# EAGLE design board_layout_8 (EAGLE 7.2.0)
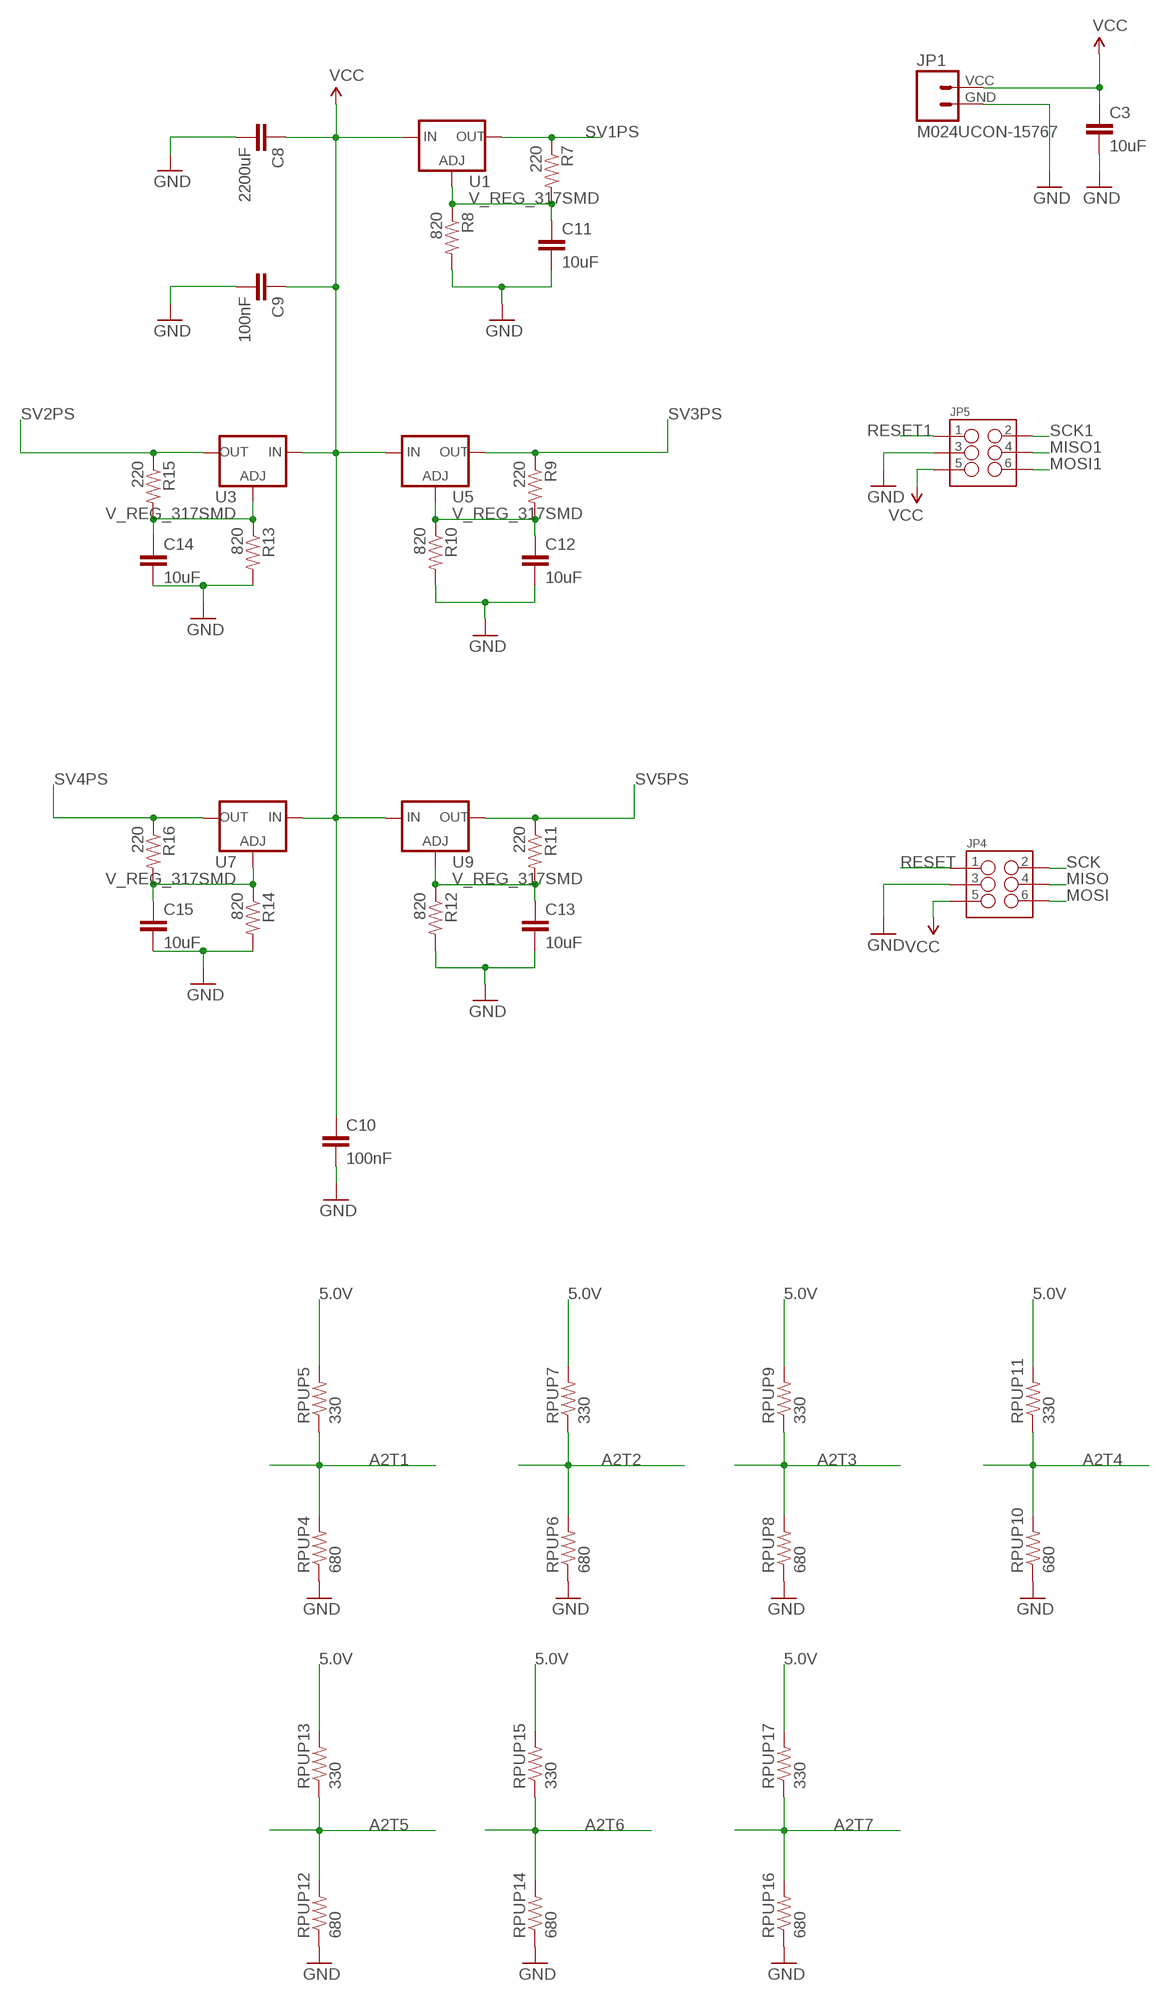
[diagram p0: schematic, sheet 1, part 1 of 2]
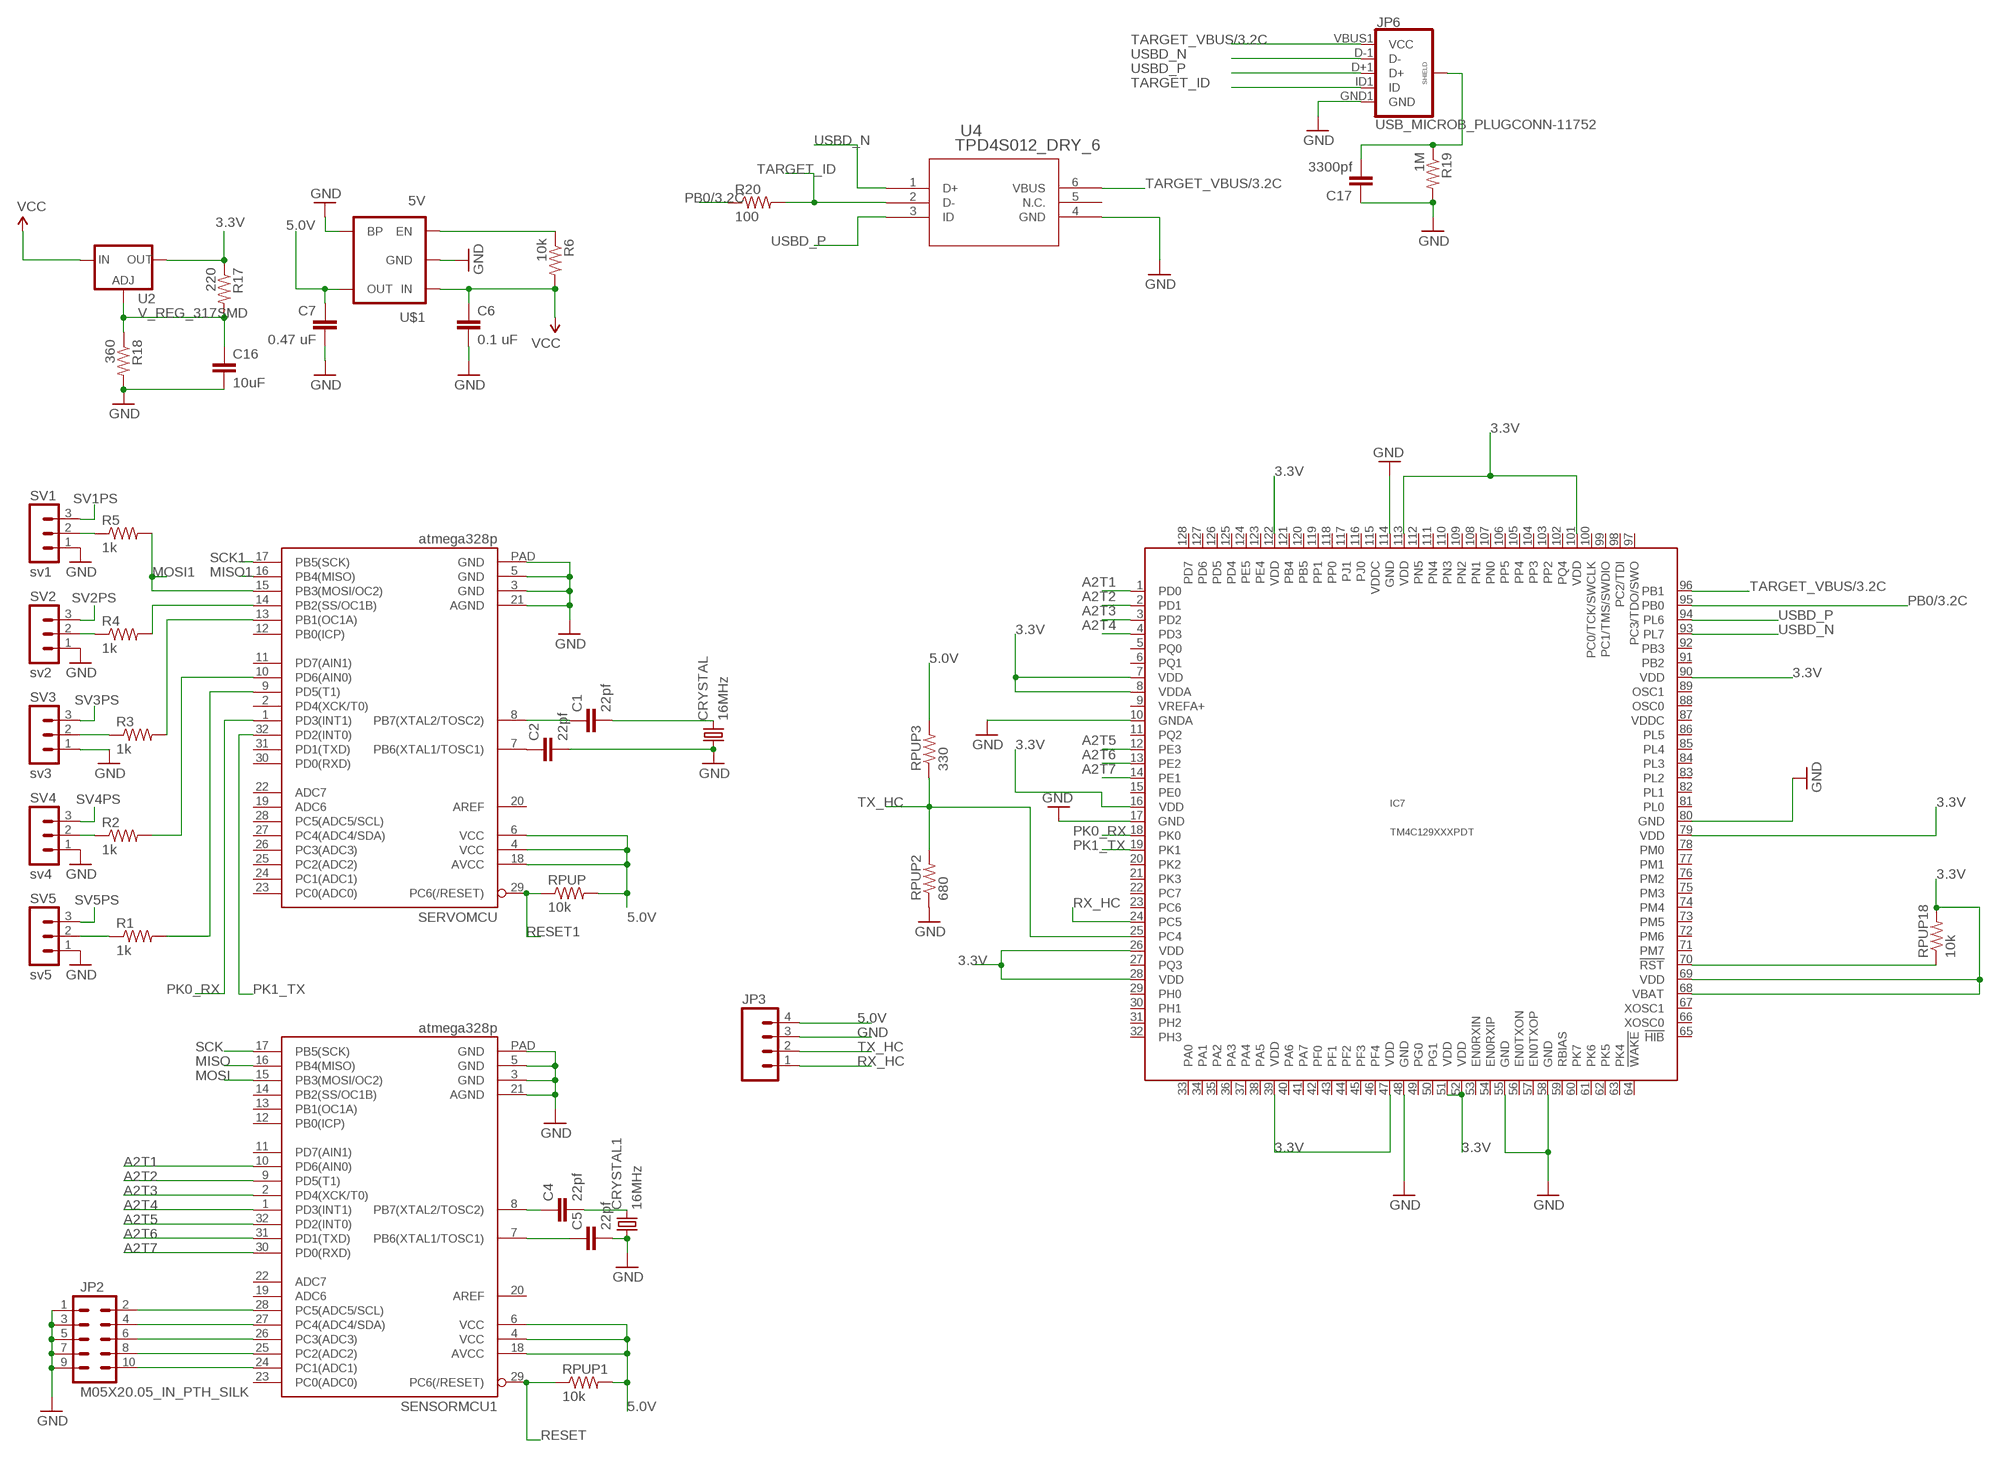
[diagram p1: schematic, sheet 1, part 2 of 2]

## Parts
C1  22pf  CAP0402-CAP  [0402-CAP]
C2  22pf  CAP0402-CAP  [0402-CAP]
C3  10uF  CAP0805  [0805]
C4  22pf  CAP0402-CAP  [0402-CAP]
C5  22pf  CAP0402-CAP  [0402-CAP]
C6  0.1 uF  CAP0805  [0805]
C7  0.47 uF  CAP0805  [0805]
C8  2200uF  CAP0805  [0805]
C9  100nF  CAP0805  [0805]
C10  100nF  CAP0805  [0805]
C11  10uF  CAP0805  [0805]
C12  10uF  CAP0805  [0805]
C13  10uF  CAP0805  [0805]
C14  10uF  CAP0805  [0805]
C15  10uF  CAP0805  [0805]
C16  10uF  CAP0805  [0805]
C17  3300pf  CAP0402-CAP  [0402-CAP]
CRYSTAL  16MHz  CRYSTALTC26V  [TC26V]
CRYSTAL1  16MHz  CRYSTALTC26V  [TC26V]
IC7  TM4C129XXXPDT  [PDT_S-PQFP-G128]
JP1  M024UCON-15767  [JST-2-SMD-VERT]
JP2  M05X20.05_IN_PTH_SILK  [2X5_PTH_SILK_.05]
JP3  M04SMD  [1X04-SMD]
JP4  M03X2  [2X3_SMD]
JP5  M03X2  [2X3_SMD]
JP6  USB_MICROB_PLUGCONN-11752  [USB-B-MICRO-SMD_V03]
R1  1k  RESISTOR0402-RES  [0402-RES]
R2  1k  RESISTOR0402-RES  [0402-RES]
R3  1k  RESISTOR0402-RES  [0402-RES]
R4  1k  RESISTOR0402-RES  [0402-RES]
R5  1k  RESISTOR0402-RES  [0402-RES]
R6  10k  RESISTOR0805-RES  [0805]
R7  220  RESISTOR0805-RES  [0805]
R8  820  RESISTOR0805-RES  [0805]
R9  220  RESISTOR0805-RES  [0805]
R10  820  RESISTOR0805-RES  [0805]
R11  220  RESISTOR0805-RES  [0805]
R12  820  RESISTOR0805-RES  [0805]
R13  820  RESISTOR0805-RES  [0805]
R14  820  RESISTOR0805-RES  [0805]
R15  220  RESISTOR0805-RES  [0805]
R16  220  RESISTOR0805-RES  [0805]
R17  220  RESISTOR0805-RES  [0805]
R18  360  RESISTOR0805-RES  [0805]
R19  1M  RESISTOR0805-RES  [0805]
R20  100  RESISTOR0805-RES  [0805]
RPUP  10k  RESISTOR0402-RES  [0402-RES]
RPUP1  10k  RESISTOR0402-RES  [0402-RES]
RPUP2  680  RESISTOR0402-RES  [0402-RES]
RPUP3  330  RESISTOR0402-RES  [0402-RES]
RPUP4  680  RESISTOR0402-RES  [0402-RES]
RPUP5  330  RESISTOR0402-RES  [0402-RES]
RPUP6  680  RESISTOR0402-RES  [0402-RES]
RPUP7  330  RESISTOR0402-RES  [0402-RES]
RPUP8  680  RESISTOR0402-RES  [0402-RES]
RPUP9  330  RESISTOR0402-RES  [0402-RES]
RPUP10  680  RESISTOR0402-RES  [0402-RES]
RPUP11  330  RESISTOR0402-RES  [0402-RES]
RPUP12  680  RESISTOR0402-RES  [0402-RES]
RPUP13  330  RESISTOR0402-RES  [0402-RES]
RPUP14  680  RESISTOR0402-RES  [0402-RES]
RPUP15  330  RESISTOR0402-RES  [0402-RES]
RPUP16  680  RESISTOR0402-RES  [0402-RES]
RPUP17  330  RESISTOR0402-RES  [0402-RES]
RPUP18  10k  RESISTOR0402-RES  [0402-RES]
SENSORMCU1  atmega328p  ATMEGA328P_MLFMLF32  [MLF32-PAD]
SERVOMCU  atmega328p  ATMEGA328P_MLFMLF32  [MLF32-PAD]
SV1  sv1  MA03-1  [MA03-1]
SV2  sv2  MA03-1  [MA03-1]
SV3  sv3  MA03-1  [MA03-1]
SV4  sv4  MA03-1  [MA03-1]
SV5  sv5  MA03-1  [MA03-1]
U1  V_REG_317SMD  [SOT223]
U2  V_REG_317SMD  [SOT223]
U3  V_REG_317SMD  [SOT223]
U4  TPD4S012_DRY_6  [DRY6]
U5  V_REG_317SMD  [SOT223]
U7  V_REG_317SMD  [SOT223]
U9  V_REG_317SMD  [SOT223]
U$1  5V  V_REG_MIC52055V  [SOT23-5]

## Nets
3.3V: IC7.7(VDD) IC7.8(VDDA) IC7.16(VDD) IC7.26(VDD) IC7.28(VDD) IC7.39(VDD) IC7.47(VDD) IC7.51(VDD) IC7.52(VDD) IC7.68(VBAT) IC7.69(VDD) IC7.79(VDD) IC7.90(VDD) IC7.101(VDD) IC7.113(VDD) IC7.122(VDD) R17.1 RPUP18.2 U2.2(OUT)
5.0V: C7.1 JP3.4 RPUP1.2 RPUP3.2 RPUP5.2 RPUP7.2 RPUP9.2 RPUP11.2 RPUP13.2 RPUP15.2 RPUP17.2 RPUP.2 SENSORMCU1.4(VCC) SENSORMCU1.6(VCC) SENSORMCU1.18(AVCC) SERVOMCU.4(VCC) SERVOMCU.6(VCC) SERVOMCU.18(AVCC) U$1.5(OUT)
A2T1: IC7.1(PD0) RPUP4.2 RPUP5.1 SENSORMCU1.10(PD6(AIN0))
A2T2: IC7.2(PD1) RPUP6.2 RPUP7.1 SENSORMCU1.9(PD5(T1))
A2T3: IC7.3(PD2) RPUP8.2 RPUP9.1 SENSORMCU1.2(PD4(XCK/T0))
A2T4: IC7.4(PD3) RPUP10.2 RPUP11.1 SENSORMCU1.1(PD3(INT1))
A2T5: IC7.12(PE3) RPUP12.2 RPUP13.1 SENSORMCU1.32(PD2(INT0))
A2T6: IC7.13(PE2) RPUP14.2 RPUP15.1 SENSORMCU1.31(PD1(TXD))
A2T7: IC7.14(PE1) RPUP16.2 RPUP17.1 SENSORMCU1.30(PD0(RXD))
GND: C2.2 C3.2 C5.2 C6.2 C7.2 C8.2 C9.2 C10.2 C11.2 C12.2 C13.2 C14.2 C15.2 C16.2 C17.1 CRYSTAL1.1 CRYSTAL.1 IC7.10(GNDA) IC7.17(GND) IC7.48(GND) IC7.55(GND) IC7.58(GND) IC7.80(GND) IC7.114(GND) JP1.GND JP2.1 JP2.3 JP2.5 JP2.7 JP2.9 JP3.3 JP4.3 JP5.3 JP6.GND1(GND) R8.2 R10.2 R12.2 R13.2 R14.2 R18.2 R19.2 RPUP2.1 RPUP4.1 RPUP6.1 RPUP8.1 RPUP10.1 RPUP12.1 RPUP14.1 RPUP16.1 SENSORMCU1.3(GND) SENSORMCU1.5(GND) SENSORMCU1.21(AGND) SENSORMCU1.PAD(GND) SERVOMCU.3(GND) SERVOMCU.5(GND) SERVOMCU.21(AGND) SERVOMCU.PAD(GND) SV1.1 SV2.1 SV3.1 SV4.1 SV5.1 U4.4(GND) U$1.2(GND) U$1.4(BP)
MISO: JP4.4 SENSORMCU1.16(PB4(MISO))
MISO1: JP5.4 SERVOMCU.16(PB4(MISO))
MOSI: JP4.6 SENSORMCU1.15(PB3(MOSI/OC2))
MOSI1: JP5.6 R5.2 SERVOMCU.15(PB3(MOSI/OC2))
N$1: R6.1 U$1.3(EN)
N$2: R4.2 SERVOMCU.14(PB2(SS/OC1B))
N$3: R3.2 SERVOMCU.13(PB1(OC1A))
N$4: C11.1 R7.2 R8.1 U1.1(ADJ)
N$5: R2.1 SV4.2
N$6: R1.1 SV5.2
N$7: R2.2 SERVOMCU.10(PD6(AIN0))
N$8: R1.2 SERVOMCU.9(PD5(T1))
N$9: R3.1 SV3.2
N$10: C1.1 SERVOMCU.8(PB7(XTAL2/TOSC2))
N$11: C2.1 SERVOMCU.7(PB6(XTAL1/TOSC1))
N$12: R5.1 SV1.2
N$13: R4.1 SV2.2
N$14: C16.1 R17.2 R18.1 U2.1(ADJ)
N$15: JP2.10 SENSORMCU1.24(PC1(ADC1))
N$16: JP2.8 SENSORMCU1.25(PC2(ADC2))
N$17: C4.1 SENSORMCU1.8(PB7(XTAL2/TOSC2))
N$18: C4.2 CRYSTAL1.2
N$19: C5.1 SENSORMCU1.7(PB6(XTAL1/TOSC1))
N$20: C1.2 CRYSTAL.2
N$21: JP2.6 SENSORMCU1.26(PC3(ADC3))
N$22: JP2.4 SENSORMCU1.27(PC4(ADC4/SDA))
N$23: JP2.2 SENSORMCU1.28(PC5(ADC5/SCL))
N$25: C12.1 R9.2 R10.1 U5.1(ADJ)
N$26: C13.1 R11.2 R12.1 U9.1(ADJ)
N$29: C14.1 R13.1 R15.2 U3.1(ADJ)
N$31: C15.1 R14.1 R16.2 U7.1(ADJ)
N$38: C17.2 JP6.SHIELD1(SHIELD) JP6.SHIELD2(SHIELD) JP6.SHIELD3(SHIELD) R19.1
N$41: IC7.70(!RST) RPUP18.1
PB0/3.2C: IC7.95(PB0) R20.1
PK0_RX: IC7.18(PK0) SERVOMCU.1(PD3(INT1))
PK1_TX: IC7.19(PK1) SERVOMCU.32(PD2(INT0))
RESET: JP4.1 RPUP1.1 SENSORMCU1.29(PC6(/RESET))
RESET1: JP5.1 RPUP.1 SERVOMCU.29(PC6(/RESET))
RX_HC: IC7.24(PC5) JP3.1
SCK: JP4.2 SENSORMCU1.17(PB5(SCK))
SCK1: JP5.2 SERVOMCU.17(PB5(SCK))
SV1PS: R7.1 SV1.3 U1.2(OUT)
SV2PS: R15.1 SV2.3 U3.2(OUT)
SV3PS: R9.1 SV3.3 U5.2(OUT)
SV4PS: R16.1 SV4.3 U7.2(OUT)
SV5PS: R11.1 SV5.3 U9.2(OUT)
TARGET_ID: JP6.ID1(ID) R20.2 U4.2(D-)
TARGET_VBUS/3.2C: IC7.96(PB1) JP6.VBUS1(VCC) U4.6(VBUS)
TX_HC: IC7.25(PC4) JP3.2 RPUP2.2 RPUP3.1
USBD_N: IC7.93(PL7) JP6.D-1(D-) U4.1(D+)
USBD_P: IC7.94(PL6) JP6.D+1(D+) U4.3(ID)
VCC: C3.1 C6.1 C8.1 C9.1 C10.1 JP1.VCC JP4.5 JP5.5 R6.2 U1.3(IN) U2.3(IN) U3.3(IN) U5.3(IN) U7.3(IN) U9.3(IN) U$1.1(IN)
Unconnected: IC7.5(PQ0) IC7.6(PQ1) IC7.9(VREFA+) IC7.11(PQ2) IC7.15(PE0) IC7.20(PK2) IC7.21(PK3) IC7.22(PC7) IC7.23(PC6) IC7.27(PQ3) IC7.29(PH0) IC7.30(PH1) IC7.31(PH2) IC7.32(PH3) IC7.33(PA0) IC7.34(PA1) IC7.35(PA2) IC7.36(PA3) IC7.37(PA4) IC7.38(PA5) IC7.40(PA6) IC7.41(PA7) IC7.42(PF0) IC7.43(PF1) IC7.44(PF2) IC7.45(PF3) IC7.46(PF4) IC7.49(PG0) IC7.50(PG1) IC7.53(EN0RXIN) IC7.54(EN0RXIP) IC7.56(EN0TXON) IC7.57(EN0TXOP) IC7.59(RBIAS) IC7.60(PK7) IC7.61(PK6) IC7.62(PK5) IC7.63(PK4) IC7.64(!WAKE) IC7.65(!HIB) IC7.66(XOSC0) IC7.67(XOSC1) IC7.71(PM7) IC7.72(PM6) IC7.73(PM5) IC7.74(PM4) IC7.75(PM3) IC7.76(PM2) IC7.77(PM1) IC7.78(PM0) IC7.81(PL0) IC7.82(PL1) IC7.83(PL2) IC7.84(PL3) IC7.85(PL4) IC7.86(PL5) IC7.87(VDDC) IC7.88(OSC0) IC7.89(OSC1) IC7.91(PB2) IC7.92(PB3) IC7.97(PC3/TDO/SWO) IC7.98(PC2/TDI) IC7.99(PC1/TMS/SWDIO) IC7.100(PC0/TCK/SWCLK) IC7.102(PQ4) IC7.103(PP2) IC7.104(PP3) IC7.105(PP4) IC7.106(PP5) IC7.107(PN0) IC7.108(PN1) IC7.109(PN2) IC7.110(PN3) IC7.111(PN4) IC7.112(PN5) IC7.115(VDDC) IC7.116(PJ0) IC7.117(PJ1) IC7.118(PP0) IC7.119(PP1) IC7.120(PB5) IC7.121(PB4) IC7.123(PE4) IC7.124(PE5) IC7.125(PD4) IC7.126(PD5) IC7.127(PD6) IC7.128(PD7) SENSORMCU1.11(PD7(AIN1)) SENSORMCU1.12(PB0(ICP)) SENSORMCU1.13(PB1(OC1A)) SENSORMCU1.14(PB2(SS/OC1B)) SENSORMCU1.19(ADC6) SENSORMCU1.20(AREF) SENSORMCU1.22(ADC7) SENSORMCU1.23(PC0(ADC0)) SERVOMCU.2(PD4(XCK/T0)) SERVOMCU.11(PD7(AIN1)) SERVOMCU.12(PB0(ICP)) SERVOMCU.19(ADC6) SERVOMCU.20(AREF) SERVOMCU.22(ADC7) SERVOMCU.23(PC0(ADC0)) SERVOMCU.24(PC1(ADC1)) SERVOMCU.25(PC2(ADC2)) SERVOMCU.26(PC3(ADC3)) SERVOMCU.27(PC4(ADC4/SDA)) SERVOMCU.28(PC5(ADC5/SCL)) SERVOMCU.30(PD0(RXD)) SERVOMCU.31(PD1(TXD)) U4.5(N.C.)

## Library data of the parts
C1 C2 C4-C7 C17 = SparkFun-Passives:CAP: Capacitor
C3 C8-C16 = SparkFun-Capacitors:CAP: Capacitor
CRYSTAL CRYSTAL1 = crystal:CRYSTAL: CRYSTAL; OC_FARNELL: unknown; OC_NEWARK: unknown
IC7 = ti-tiva:TM4C129XXX
JP1 = SparkFun-Connectors:M02: Standard 2-pin 0.1" header. Use with
JP2 = SparkFun-Connectors:M05X2: Header 5x2 Standard 10-pin dual row 0.1" header. Commonly used with AVR-ISP. Use with Spark Fun Electronics SKU: PRT-00778
JP3 = SparkFun-Connectors:M04: Header 4 Standard 4-pin 0.1" header. Use with straight break away headers (SKU : PRT-00116), right angle break away headers (PRT-00553), swiss pins (PRT-00743), machine pins (PRT-00117), and female headers (PRT-00115). Molex polarized connector foot print use with SKU : PRT-08231 with associated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
JP4 JP5 = SparkFun-Connectors:M03X2: 2x3 .1" header. Shrouded, with keying- CONN-10681 SMT- CONN-11415 Pogo pins- HW-11044; PROD_ID: CONN-11290
JP6 = SparkFun-Connectors:USB_MICROB_PLUG: USB Micro-B connectors Some male, some female. Watch your step!; PROD_ID: CONN-11752
R1-R20 RPUP RPUP1-RPUP18 = SparkFun-Passives:RESISTOR: Resistor
SENSORMCU1 SERVOMCU = SparkFun-DigitalIC:ATMEGA328P_MLF: 32-Pin Atmega328 part Commonly used on Arduino compatible boards Available in QFP and QFN packages TQFP is IC-09069 QFN is non-stock
SV1-SV5 = con-lstb:MA03-1: PIN HEADER; OC_FARNELL: unknown; OC_NEWARK: unknown
U1-U3 U5 U7 U9 = SparkFun-PowerIC:V_REG_317: Voltage Regulator Standard LM317 adjustable voltage regulator. AOI (Adjust Output Input). Google 'LM317 Calculator' for easy to use app to get the two resistor values needed. 240/720 for 5V output. 240/390 for 3.3V output. Spark Fun Electronics SKU : COM-00527
U4 = esd_tp:TPD4S012_DRY_6; DATASHEETURL: http://www.ti.com/lit/gpn/TPD4S012; DESCRIPTION: 4-Channel USB ESD Solution with Power Clamp; FAMILY_NAME: ESD Solution; GENERIC_PART_NUMBER: TPD4S012; INDUSTRY_STD_PKG_TYPE: SON; MANUFACTURER: Texas Instruments; MANUFACTURER_PART_NUMBER: tpd4s012_dry_6; PACKAGE_DESIGNATOR: DRY; PIN_COUNT: 6; VENDOR: Texas Instruments
U$1 = SparkFun-PowerIC:V_REG_MIC5205: V_REG MIC5219 Standard 3.3V and 5V 150mA LDO voltage regulator in SOT-23 layout. Micrel part MIC5205. BP (by-pass) pin is used to lower output noise with 470pF cap, may be left open.; PROD_ID: VREG-00823

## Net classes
0 default: clearance 0.06 mm

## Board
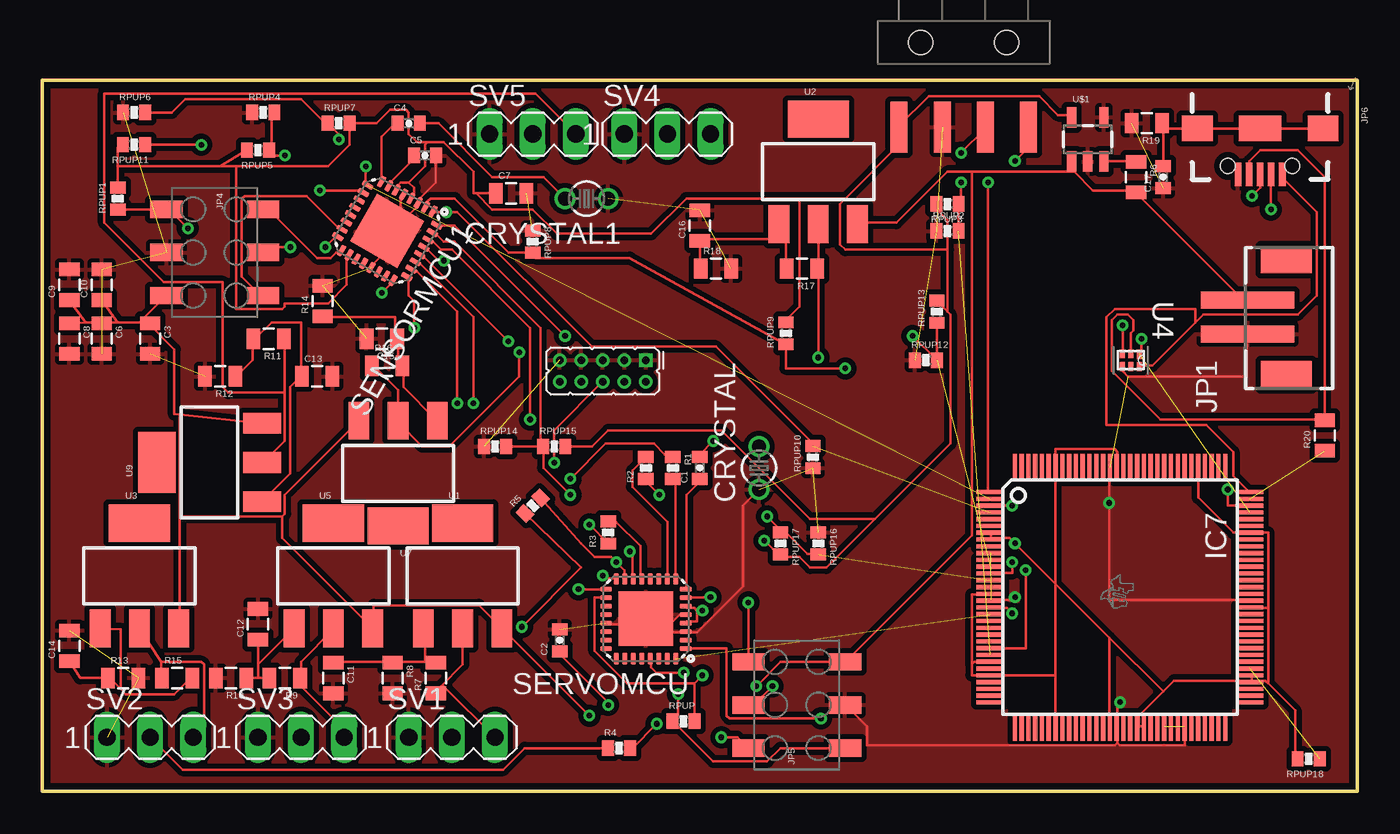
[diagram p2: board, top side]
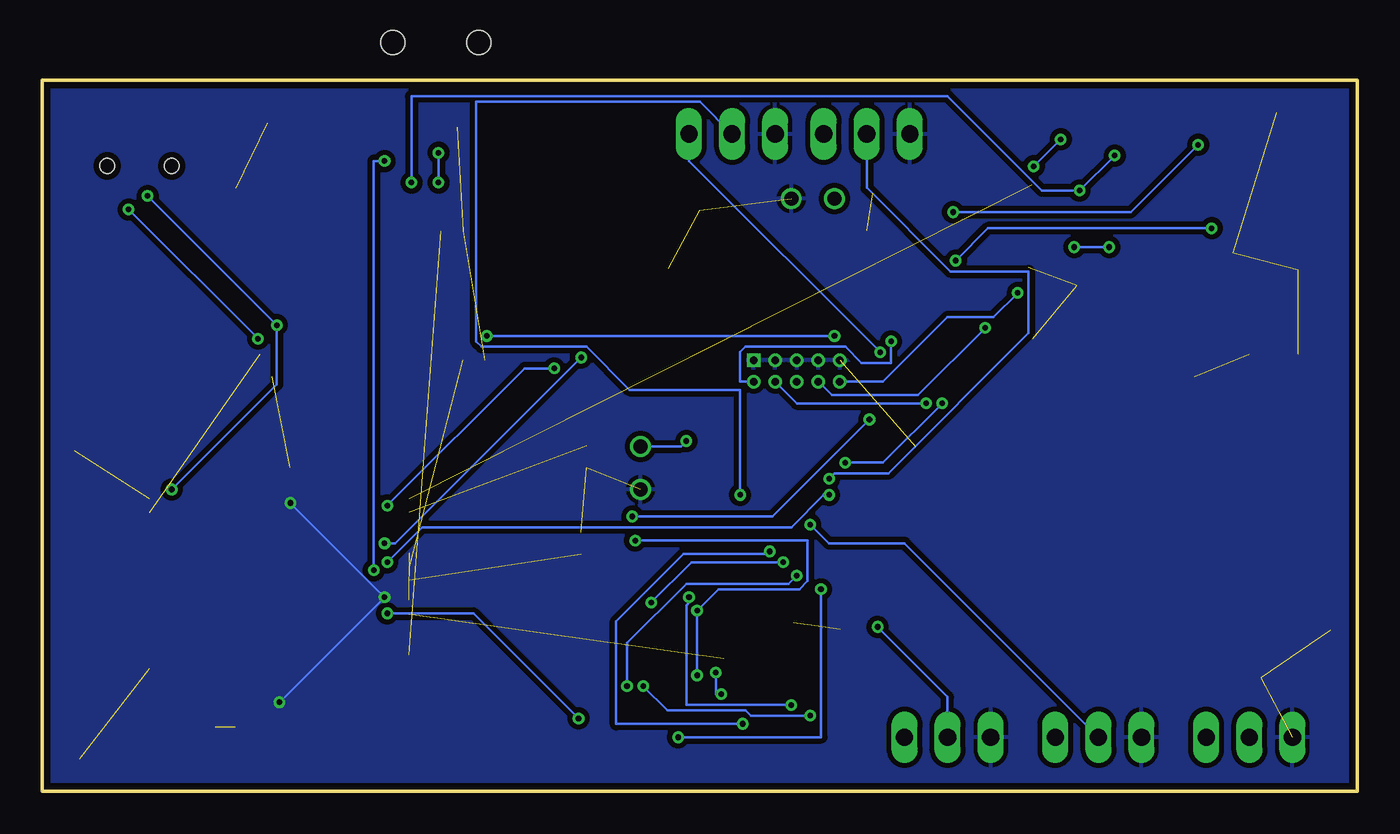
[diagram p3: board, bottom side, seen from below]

Size 77.47 x 41.91 mm. Coordinates in mm from the lower left corner, seen from the top.
Outline: 0,0 0,41.91 77.47,41.91 77.47,0 0,0
Copper layers (1*16): Top 0.0356mm / dielectric 1.5011mm / Bottom 0.0356mm
Design rules "PCB_order": minimum track width 6mil, minimum drill 13mil, track to track 6mil, track to pad 6mil, pad to pad 6mil, via to via 6mil, smd to smd 6mil, copper to edge 15mil, drill to drill 6mil, minimum pad ring 7mil, minimum via ring 7mil, stop-mask expansion 3mil, vias tented up to drill 0mil, thermal gap 10mil

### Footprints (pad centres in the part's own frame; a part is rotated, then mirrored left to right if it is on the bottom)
0402-CAP = smd 0.7 x 0.9: 1 -0.65,0; 2 0.65,0
0805 = smd 0.8 x 1.2: 1 -0.9,0; 2 0.9,0
TC26V = drill 0.813: 1 -1.27,0; 2 1.27,0
PDT_S-PQFP-G128 = smd 0.25 x 1.6: 1 -6.2,-7.65; 2 -5.8,-7.65; 3 -5.4,-7.65; 4 -5,-7.65; 5 -4.6,-7.65; 6 -4.2,-7.65; 7 -3.8,-7.65; 8 -3.4,-7.65; 9 -3,-7.65; 10 -2.6,-7.65; 11 -2.2,-7.65; 12 -1.8,-7.65; 13 -1.4,-7.65; 14 -1,-7.65; 15 -0.6,-7.65; 16 -0.2,-7.65; 17 0.2,-7.65; 18 0.6,-7.65; 19 1,-7.65; 20 1.4,-7.65; 21 1.8,-7.65; 22 2.2,-7.65; 23 2.6,-7.65; 24 3,-7.65; 25 3.4,-7.65; 26 3.8,-7.65; 27 4.2,-7.65; 28 4.6,-7.65; 29 5,-7.65; 30 5.4,-7.65; 31 5.8,-7.65; 32 6.2,-7.65; 65 6.2,7.65; 66 5.8,7.65; 67 5.4,7.65; 68 5,7.65; 69 4.6,7.65; 70 4.2,7.65; 71 3.8,7.65; 72 3.4,7.65; 73 3,7.65; 74 2.6,7.65; 75 2.2,7.65; 76 1.8,7.65; 77 1.4,7.65; 78 1,7.65; 79 0.6,7.65; 80 0.2,7.65; 81 -0.2,7.65; 82 -0.6,7.65; 83 -1,7.65; 84 -1.4,7.65; 85 -1.8,7.65; 86 -2.2,7.65; 87 -2.6,7.65; 88 -3,7.65; 89 -3.4,7.65; 90 -3.8,7.65; 91 -4.2,7.65; 92 -4.6,7.65; 93 -5,7.65; 94 -5.4,7.65; 95 -5.8,7.65; 96 -6.2,7.65 | smd 1.6 x 0.25: 33 7.65,-6.2; 34 7.65,-5.8; 35 7.65,-5.4; 36 7.65,-5; 37 7.65,-4.6; 38 7.65,-4.2; 39 7.65,-3.8; 40 7.65,-3.4; 41 7.65,-3; 42 7.65,-2.6; 43 7.65,-2.2; 44 7.65,-1.8; 45 7.65,-1.4; 46 7.65,-1; 47 7.65,-0.6; 48 7.65,-0.2; 49 7.65,0.2; 50 7.65,0.6; 51 7.65,1; 52 7.65,1.4; 53 7.65,1.8; 54 7.65,2.2; 55 7.65,2.6; 56 7.65,3; 57 7.65,3.4; 58 7.65,3.8; 59 7.65,4.2; 60 7.65,4.6; 61 7.65,5; 62 7.65,5.4; 63 7.65,5.8; 64 7.65,6.2; 97 -7.65,6.2; 98 -7.65,5.8; 99 -7.65,5.4; 100 -7.65,5; 101 -7.65,4.6; 102 -7.65,4.2; 103 -7.65,3.8; 104 -7.65,3.4; 105 -7.65,3; 106 -7.65,2.6; 107 -7.65,2.2; 108 -7.65,1.8; 109 -7.65,1.4; 110 -7.65,1; 111 -7.65,0.6; 112 -7.65,0.2; 113 -7.65,-0.2; 114 -7.65,-0.6; 115 -7.65,-1; 116 -7.65,-1.4; 117 -7.65,-1.8; 118 -7.65,-2.2; 119 -7.65,-2.6; 120 -7.65,-3; 121 -7.65,-3.4; 122 -7.65,-3.8; 123 -7.65,-4.2; 124 -7.65,-4.6; 125 -7.65,-5; 126 -7.65,-5.4; 127 -7.65,-5.8; 128 -7.65,-6.2
JST-2-SMD-VERT = smd 1 x 5.5: GND 1,-2; VCC -1,-2 | smd 1.6 x 3: P$1 -3.4,0.27; P$2 3.4,0.27
2X5_PTH_SILK_.05 = drill 0.432 square: 1 0,6.35 | drill 0.432: 2 1.27,6.35; 3 0,5.08; 4 1.27,5.08; 5 0,3.81; 6 1.27,3.81; 7 0,2.54; 8 1.27,2.54; 9 0,1.27; 10 1.27,1.27
1X04-SMD = smd 1 x 3: 1 -3.81,5; 2 -1.27,5; 3 1.27,5; 4 3.81,5 | hole 1.4: -2.54,0; 2.54,0
2X3_SMD = smd 1.02 x 1.9: 1 -2.54,-2.85; 2 -2.54,2.85; 3 0,-2.85; 4 0,2.85; 5 2.54,-2.85; 6 2.54,2.85
USB-B-MICRO-SMD_V03 = smd 1.4 x 0.4: D+1 2.7,0; D-1 2.7,0.65; GND1 2.7,-1.3; ID1 2.7,-0.65; VBUS1 2.7,1.3 | smd 1.5 x 1.8: SHIELD1 0,3.7; SHIELD2 0,-3.7 | smd 1.5 x 2.5: SHIELD3 0,0 | hole 0.85: 2.2,1.9; 2.2,-1.9
0402-RES = smd 0.7 x 0.9: 1 -0.65,0; 2 0.65,0
MLF32-PAD = smd 0.7 x 0.3: 1 -2.35,1.75; 2 -2.35,1.25; 3 -2.35,0.75; 4 -2.35,0.25; 5 -2.35,-0.25; 6 -2.35,-0.75; 7 -2.35,-1.25; 8 -2.35,-1.75; 17 2.35,-1.75; 18 2.35,-1.25; 19 2.35,-0.75; 20 2.35,-0.25; 21 2.35,0.25; 22 2.35,0.75; 23 2.35,1.25; 24 2.35,1.75 | smd 0.3 x 0.7: 9 -1.75,-2.35; 10 -1.25,-2.35; 11 -0.75,-2.35; 12 -0.25,-2.35; 13 0.25,-2.35; 14 0.75,-2.35; 15 1.25,-2.35; 16 1.75,-2.35; 25 1.75,2.35; 26 1.25,2.35; 27 0.75,2.35; 28 0.25,2.35; 29 -0.25,2.35; 30 -0.75,2.35; 31 -1.25,2.35; 32 -1.75,2.35 | smd 3.2 x 3.2: PAD 0,0
MA03-1 = drill 1.016 long: 1 -2.54,0; 2 0,0; 3 2.54,0
SOT223 = smd 1.219 x 2.235: 1 -2.311,-3.099; 2 0,-3.099; 3 2.311,-3.099 | smd 3.6 x 2.2: 4 0,3.099
DRY6 = smd 0.559 x 0.305: 1 -0.355,0.5 | smd 0.508 x 0.305: 2 -0.37,0; 3 -0.37,-0.5; 4 0.37,-0.5; 5 0.37,0; 6 0.37,0.5
SOT23-5 = smd 0.55 x 1.2: 1 -0.95,-1.3; 2 0,-1.3; 3 0.95,-1.3; 4 0.95,1.3; 5 -0.95,1.3

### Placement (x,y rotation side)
C1  38.74,19.05 90 top
C2  30.48,8.89 90 top
C3  6.35,26.67 270 top
C4  21.59,39.37 0 top
C5  22.54,37.47 0 top
C6  3.49,26.67 270 top
C7  27.62,35.24 0 top
C8  1.59,26.67 270 top
C9  1.59,29.84 90 top
C10  3.49,29.84 90 top
C11  17.14,6.67 270 top
C12  12.7,9.84 90 top
C13  16.19,24.45 0 top
C14  1.59,8.57 90 top
C15  20,26.67 180 top
C16  38.74,33.34 90 top
C17  66.04,36.2 90 top
CRYSTAL  42.23,19.05 90 top
CRYSTAL1  32.07,34.92 180 top
IC7  63.5,11.43 270 top
JP1  73.02,27.94 270 top
JP2  29.21,25.4 270 top
JP3  54.29,44.13 180 top
JP4  10.16,31.75 270 top
JP5  44.45,5.08 90 top
JP6  71.75,39.05 270 top
R1  37.15,19.05 270 top
R2  35.56,19.05 90 top
R3  33.34,15.24 90 top
R4  33.97,2.54 0 top
R5  28.89,16.83 45 top
R6  64.45,36.2 270 top
R7  23.18,6.67 90 top
R8  20.64,6.67 270 top
R9  14.29,6.67 180 top
R10  11.11,6.67 180 top
R11  13.33,26.67 180 top
R12  10.48,24.45 180 top
R13  4.76,6.67 0 top
R14  16.51,28.89 90 top
R15  7.94,6.67 0 top
R16  20.32,25.08 0 top
R17  44.77,30.8 180 top
R18  39.69,30.8 0 top
R19  65.09,39.37 180 top
R20  75.56,20.95 90 top
RPUP  37.78,4.13 0 top
RPUP1  4.45,34.92 90 top
RPUP2  53.34,33.02 0 top
RPUP3  53.34,34.61 180 top
RPUP4  13.02,40.01 0 top
RPUP5  12.7,37.78 180 top
RPUP6  5.4,40.01 0 top
RPUP7  17.46,39.37 0 top
RPUP8  28.89,32.38 270 top
RPUP9  43.82,26.99 90 top
RPUP10  45.4,19.68 90 top
RPUP11  5.4,38.1 180 top
RPUP12  52.07,25.4 0 top
RPUP13  52.71,28.26 90 top
RPUP14  26.67,20.32 0 top
RPUP15  30.16,20.32 0 top
RPUP16  45.72,14.61 270 top
RPUP17  43.5,14.61 270 top
RPUP18  74.61,1.91 180 top
SENSORMCU1  20.32,33.02 240 top
SERVOMCU  35.56,10.16 180 top
SV1  24.13,3.17 0 top
SV2  6.35,3.17 0 top
SV3  15.24,3.17 0 top
SV4  36.83,38.73 0 top
SV5  28.89,38.73 0 top
U1  24.77,12.7 0 top
U2  45.72,36.51 0 top
U3  5.71,12.7 0 top
U4  64.14,25.4 270 top
U5  17.14,12.7 0 top
U7  20.95,18.73 180 top
U9  9.84,19.37 90 top
U$1  61.6,38.42 0 top

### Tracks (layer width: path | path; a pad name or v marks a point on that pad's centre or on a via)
3.3V  (via drill 0.33)
  Top 0.152: U2.2 45.72,30.8 | 72.23,6.35 72.07,6.51 71.28,6.51 | 72.23,6.35 73.82,4.76 73.82,1.91 RPUP18.2 | 64.61,3.81 64.61,4.45 66.04,5.87 | 66.04,5.87 66.67,6.51 71.12,6.51 IC7.68 71.28,6.51 | 55.88,14.92 56.99,14.92 v57.31,14.61 59.69,12.22 | 66.04,5.87 62.87,9.05 | 62.87,9.05 59.69,12.22 | v45.72,25.56 45.72,30.8 | 45.72,30.8 R17.1 | 54.77,7.46 54.77,6.83 55.72,6.83 IC7.28 55.88,6.83 59.69,6.83 | 54.77,7.46 54.93,7.62 55.72,7.62 IC7.26 | 54.77,7.46 54.77,11.59 55.72,11.59 IC7.16 | 55.88,14.92 55.88,15.24 IC7.7 | 55.88,14.92 IC7.8 | 64.61,3.81 64.93,3.81 IC7.52 | 64.61,3.81 IC7.51 | 59.69,12.22 59.69,6.83 | 59.69,6.83 59.69,3.81 IC7.39 | 59.69,12.22 59.69,19.05 IC7.122 59.69,19.21 59.69,20.16 63.18,20.16 63.34,20 63.34,19.21 IC7.113 | 62.87,9.05 62.87,3.81 IC7.47 | 71.28,6.51 71.28,6.83 IC7.69 | 72.23,10.79 71.28,10.79 IC7.79 | 72.23,6.35 72.23,10.79 | 72.23,10.79 72.23,15.24 71.28,15.24 IC7.90 71.12,15.24 70.17,15.24 68.1,17.3 68.1,19.05 IC7.101
  Bottom 0.152: v45.72,25.56 56.67,14.61 v57.31,14.61
5.0V  (via drill 0.33)
  Top 0.152: 4.45,36.83 4.45,37.94 4.6,38.1 RPUP11.2 | 4.45,36.83 RPUP1.2 | 4.45,36.83 10.48,36.83 | 10.48,36.83 11.43,36.83 | 11.43,36.83 16.83,36.83 18.1,38.1 18.1,39.37 RPUP7.2 19.68,39.37 20.48,40.16 21.43,40.16 21.59,40.01 21.59,38.73 22.07,38.26 22.7,38.26 | 10.48,36.83 RPUP5.2 | 21.59,35.88 21.11,35.88 20.95,35.72 20.95,35.56 SENSORMCU1.6 | 21.59,35.88 21.91,35.56 21.91,35.24 21.75,35.08 SENSORMCU1.4 | 25.56,35.24 26.51,34.29 28.89,34.29 30.32,32.86 35.88,32.86 37.94,34.92 44.61,34.92 | 25.56,35.24 C7.1 | 21.59,35.88 22.54,36.83 22.54,38.1 22.7,38.26 | 22.7,38.26 23.65,38.26 25.4,36.51 25.4,35.24 25.56,35.24 | U$1.5 60.64,39.85 59.85,39.85 58.74,40.96 52.23,40.96 50.48,39.21 JP3.4 50.48,38.1 47.31,34.92 | 43.5,13.81 44.61,13.81 45.24,13.18 46.2,13.18 49.05,16.03 | 49.05,16.03 53.5,20.48 53.5,28.1 53.34,28.26 | 53.34,28.26 52.71,28.89 RPUP13.2 | 53.34,28.26 53.34,31.91 | 53.34,31.91 53.34,33.66 52.71,34.29 52.71,34.61 RPUP3.2 | 47.31,34.92 46.99,34.61 46.99,32.23 47.31,31.91 53.34,31.91 | 47.31,34.92 44.61,34.92 | RPUP15.2 32.38,20.32 33.34,21.27 40.01,21.27 45.24,16.03 49.05,16.03 | 38.58,10.64 38.58,10 37.94,10 SERVOMCU.4 | 38.58,10.64 38.42,10.79 37.94,10.79 SERVOMCU.6 | 38.42,6.35 34.45,6.35 32.54,8.26 32.54,11.43 33.18,11.43 SERVOMCU.18 | 38.42,6.35 38.42,4.13 RPUP.2 | v38.89,10.64 38.58,10.64 | 38.42,6.35 v38.89,6.83 | 44.61,34.92 44.61,28.57 43.82,27.78 RPUP9.2 | 11.43,36.83 11.43,28.42 14.13,28.42 14.29,28.57 14.29,28.73 16.83,28.73 17.94,29.84 17.94,31.59 SENSORMCU1.18 | 43.5,13.81 v42.55,14.76 | 43.5,13.81 RPUP17.2
  Bottom 0.152: v38.89,6.83 v38.89,10.64 37.62,11.91 32.86,11.91 32.38,12.38 32.38,14.76 v42.55,14.76
A2T1  (via drill 0.33)
  Top 0.152: v16.35,35.4 18.89,35.4 SENSORMCU1.10 | v14.29,37.47 13.49,37.47 13.49,37.78 | 13.49,37.78 13.49,39.85 13.65,40.01 RPUP4.2 | 13.49,37.78 RPUP5.1 | v55.72,35.88 55.72,17.62 IC7.1
  Bottom 0.152: v14.29,37.47 v16.35,35.4 18.57,35.4 24.13,40.96 55.72,40.96 v55.72,35.88
A2T2  (via drill 0.33)  (1 unrouted)
  Top 0.152: v19.05,36.83 19.05,35.72 SENSORMCU1.9 | v17.46,38.42 17.46,38.73 16.83,39.37 RPUP7.1 16.67,39.37 15.24,40.8 8.41,40.8 7.62,40.01 RPUP6.2
  Bottom 0.152: v17.46,38.42 v19.05,36.83
A2T3  (via drill 0.33)
  Top 0.152: SENSORMCU1.2 22.54,34.45 22.7,34.61 22.7,34.77 22.86,34.92 24.29,34.92 27.46,31.75 28.89,31.75 RPUP8.2 28.89,31.59 29.05,31.43 34.61,31.43 RPUP9.1 43.82,24.92 v47.31,24.92 | v57.15,16.83 55.88,16.83 IC7.3
  Bottom 0.152: v57.15,16.83 49.05,24.92 v47.31,24.92
A2T4  (via drill 0.33)  (1 unrouted)
  Top 0.152: SENSORMCU1.1 23.02,34.13 v23.81,34.13 24.45,34.13 32.38,26.19 39.69,26.19 45.4,20.48 RPUP10.2 | v9.37,38.1 RPUP11.1
  Bottom 0.152: v9.37,38.1 13.33,34.13 v23.81,34.13
A2T5  (via drill 0.33)  (1 unrouted)
  Top 0.152: v30.8,26.83 24.29,33.34 23.34,33.34 SENSORMCU1.32 | 52.71,25.4 v51.28,26.83 | 52.71,25.4 RPUP13.1 | 52.71,25.4 RPUP12.2
  Bottom 0.152: v51.28,26.83 v30.8,26.83
A2T6  (via drill 0.33)
  Top 0.152: 29.37,20.32 29.37,27.3 24.29,32.38 23.65,32.38 23.18,32.86 23.02,32.86 SENSORMCU1.31 | 29.37,20.32 RPUP14.2 | 29.37,20.32 RPUP15.1 29.53,20.32 29.53,19.05 v31.11,17.46 | v57.15,13.49 57.15,12.86 55.88,12.86 IC7.13
  Bottom 0.152: v57.15,13.49 55.09,15.56 33.34,15.56 31.43,17.46 v31.11,17.46
A2T7  (via drill 0.33)  (1 unrouted)
  Top 0.152: v28.73,21.91 28.73,27.3 24.13,31.91 23.5,31.91 23.02,32.38 22.86,32.38 SENSORMCU1.30 | v42.7,16.19 43.5,15.4 RPUP17.1 43.5,15.24 43.82,15.24 45.09,13.97 RPUP16.2
  Bottom 0.152: v28.73,21.91 34.45,16.19 v42.7,16.19
GND  (via drill 0.33)  (21 unrouted)
  Top 0.152: SERVOMCU.PAD 35.24,9.84 33.34,9.84 SERVOMCU.21 | 36.51,9.37 36.35,9.37 SERVOMCU.PAD | 36.51,9.37 37.78,9.37 SERVOMCU.3 37.94,9.37 38.58,9.37 41.28,12.06 41.28,16.83 CRYSTAL.1 | 36.51,9.37 37.62,10.48 37.78,10.48 SERVOMCU.5 | 36.51,9.37 SERVOMCU.PAD | 20.32,32.7 20.32,31.91 19.37,30.96 SENSORMCU1.21 | 20.32,32.7 21.11,33.5 | 21.11,33.5 22.07,34.45 22.07,34.61 SENSORMCU1.3 22.22,34.77 22.22,34.92 23.18,35.88 23.18,37.47 C5.2 | 20.32,32.7 SENSORMCU1.PAD 21.11,33.5 | 21.11,33.5 21.11,34.92 21.27,35.08 SENSORMCU1.5 | v57.31,11.43 57.31,11.27 55.88,11.27 IC7.17 | IC7.114 62.87,19.05 v62.87,16.99 62.87,11.27 71.12,11.27 IC7.80 | U4.4 63.66,24.92 63.66,24.77 63.98,24.45 70.96,24.45 70.96,26.83 JP1.GND | 63.34,2.86 63.34,3.65 IC7.48 63.34,3.81 63.34,5.08 v63.5,5.24 | 63.34,2.86 63.5,2.7 67.31,2.7 67.31,3.65 IC7.58 | 63.34,2.86 63.18,2.7 48.58,2.7 48.58,3.81 JP5.3 | 28.42,35.24 C7.2
  Bottom 0.152: JP2.1 | v62.87,16.99 v57.31,11.43 v63.5,5.24
  pour Top (isolate 0.305): 0,41.91 77.47,41.91 77.47,0 0,0
  pour Bottom (isolate 0.305): 0,0 0,41.91 77.47,41.91 77.47,0
MISO  (via drill 0.33)
  Top 0.152: v16.67,32.07 17.3,32.7 SENSORMCU1.16 | v14.61,32.07 13.33,32.07 JP4.4
  Bottom 0.152: v14.61,32.07 v16.67,32.07
MISO1  (via drill 0.33)
  Top 0.152: v33.02,12.7 33.18,12.54 33.81,12.54 SERVOMCU.16 | v43.02,6.19 41.91,5.08 JP5.4
  Bottom 0.152: v33.02,12.7 33.5,12.22 39.53,12.22 43.02,8.73 v43.02,6.19
MOSI
  Top 0.152: SENSORMCU1.15 17.62,33.18 17.46,33.18 15.56,35.08 11.91,35.08 11.75,34.92 11.75,30.32 12.86,29.21 JP4.6
MOSI1  (via drill 0.33)
  Top 0.152: SERVOMCU.15 34.29,12.54 34.29,13.02 v33.81,13.49 33.5,13.81 32.54,13.81 31.75,14.61 R5.2 | v41.59,11.11 JP5.6
  Bottom 0.152: v41.59,11.11 39.21,13.49 v33.81,13.49
N$1
  Top 0.152: R6.1 64.45,37.15 62.55,37.15 U$1.3
N$2  (via drill 0.33)
  Top 0.152: v34.61,14.13 34.77,13.97 34.77,12.54 SERVOMCU.14 | v36.2,3.97 34.77,2.54 R4.2
  Bottom 0.152: v34.61,14.13 34.77,13.97 39.69,13.97 43.66,10 43.66,3.97 v36.2,3.97
N$3
  Top 0.152: SERVOMCU.13 35.24,12.54 35.24,14.45 33.81,15.88 33.34,15.88 R3.2
N$4
  Top 0.152: 20.64,7.62 17.14,7.62 C11.1 | 20.64,7.62 22.54,7.62 | 22.54,7.62 23.18,7.62 R7.2 | 20.64,7.62 R8.1 | 22.54,7.62 22.54,9.53 U1.1
N$5  (via drill 0.33)
  Top 0.152: v36.35,17.46 35.56,18.26 R2.1
  Bottom 0.152: v36.35,17.46 36.35,23.65 42.86,23.65 45.4,26.19 51.59,26.19 51.91,26.51 51.91,40.64 38.74,40.64 SV4.2
N$6  (via drill 0.33)
  Top 0.152: v31.11,18.41 33.18,20.48 36.04,20.48 36.67,19.84 37.15,19.84 R1.1
  Bottom 0.152: v31.11,18.41 30.8,18.73 27.62,18.73 19.37,26.99 19.37,30.64 23.97,30.64 28.89,35.56 SV5.2
N$7
  Top 0.152: SERVOMCU.10 36.83,12.54 36.83,15.88 34.77,17.94 34.77,18.89 35.56,19.68 R2.2
N$8
  Top 0.152: SERVOMCU.9 37.31,12.54 37.31,18.1 37.15,18.26 R1.2
N$9  (via drill 0.33)
  Top 0.152: v32.23,15.72 33.34,14.61 R3.1
  Bottom 0.152: v32.23,15.72 31.11,14.61 26.67,14.61 SV3.2
N$10
  Top 0.152: SERVOMCU.8 37.94,11.91 37.94,17.46 38.74,18.26 C1.1
N$11  (via drill 0.33)
  Top 0.152: v39.37,11.43 37.94,11.43 SERVOMCU.7 | v33.34,5.08 33.34,5.24 30.48,8.1 C2.1
  Bottom 0.152: v39.37,11.43 39.37,11.11 39.53,10.95 39.53,5.08 v33.34,5.08
N$12  (via drill 0.33)
  Top 0.152: v28.26,9.68 31.75,13.18 R5.1
  Bottom 0.152: v28.26,9.68 24.13,5.56 SV1.2
N$13
  Top 0.152: R4.1 28.42,2.54 27.15,1.27 8.26,1.27 SV2.2
N$14
  Top 0.152: R18.1 38.74,30.8 C16.1 38.74,32.54 43.82,32.54 | 43.82,32.54 43.82,33.02 43.5,33.34 U2.1 43.82,32.54 | 43.82,32.54 43.82,30.8 R17.2
N$15  (via drill 0.33)
  Top 0.152: v20,29.37 20.64,30 SENSORMCU1.24
  Bottom 0.152: v20,29.37 21.43,27.94 24.13,27.94 27.94,24.13 JP2.10
N$16  (via drill 0.33)
  Top 0.152: SENSORMCU1.25 21.59,30.32 21.59,29.21 21.91,28.89 v21.91,27.3
  Bottom 0.152: v21.91,27.3 25.88,23.34 30.96,23.34 JP2.8
N$17
  Top 0.152: SENSORMCU1.8 20,36.04 20,38.58 20.8,39.37 C4.1
N$18
  Top 0.152: C4.2 23.34,39.37 26.51,36.2 29.53,36.2 CRYSTAL1.2
N$19
  Top 0.152: SENSORMCU1.7 20.48,35.72 20.48,35.88 21.75,37.15 21.75,37.47 C5.1
N$20  (via drill 0.33)
  Top 0.152: v39.53,20.64 38.74,19.84 C1.2
  Bottom 0.152: v39.53,20.64 39.85,20.32 CRYSTAL.2
N$21  (via drill 0.33)
  Top 0.152: v24.45,22.86 24.45,28.26 22.07,30.64 21.91,30.64 21.75,30.8 SENSORMCU1.26 | v30.16,19.37 30.16,21.27 JP2.6
  Bottom 0.152: v24.45,22.86 27.94,19.37 v30.16,19.37
N$22  (via drill 0.33)
  Top 0.152: v25.4,22.86 25.4,27.94 22.22,31.11 22.07,31.11 SENSORMCU1.27
  Bottom 0.152: v25.4,22.86 33.02,22.86 JP2.4
N$23  (via drill 0.33)
  Top 0.152: v27.46,26.51 22.38,31.59 SENSORMCU1.28
  Bottom 0.152: v27.46,26.51 27.46,25.24 29.21,25.24 30.16,26.19 36.04,26.19 36.35,25.88 36.35,24.13 JP2.2
N$25
  Top 0.152: R9.2 12.7,6.67 | 12.7,6.67 R10.1 | 12.7,6.67 12.7,7.46 | 12.7,7.46 C12.1 | 12.7,7.46 14.76,9.53 U5.1
N$26
  Top 0.152: R12.1 11.43,24.45 12.38,25.4 12.38,26.67 R11.2 12.54,26.67 13.49,27.62 15.24,27.62 15.24,24.45 | 15.24,24.45 14.61,23.81 14.61,18.73 13.02,17.14 U9.1 | 15.24,24.45 C13.1
N$29
  Top 0.152: C14.1 2.22,6.67 R13.1 3.97,6.67 4.6,6.03 | 4.6,6.03 4.92,5.71 7.78,5.71 8.73,6.67 R15.2 | 4.6,6.03 4.6,9.53 U3.1
N$31
  Top 0.152: R14.1 16.51,27.94 20.8,27.94 20.8,26.67 C15.1 20.95,26.67 20.95,25.24 21.11,25.08 R16.2 21.27,25.08 21.27,23.81 23.18,21.91 U7.1
N$38
  Top 0.152: 66.04,39.05 66.04,39.37 R19.1 66.04,39.05 | 66.04,39.05 C17.2 | 66.04,39.05 JP6.SHIELD2 JP6.SHIELD3 JP6.SHIELD1
N$41  (1 unrouted)
PB0/3.2C  (1 unrouted)
PK0_RX  (via drill 0.33)
  Top 0.152: v45.88,4.29 40.48,4.29 40.32,4.45 40.32,8.41 37.94,8.41 SERVOMCU.1 | v57.15,10.48 56.83,10.79 55.88,10.79 IC7.18
  Bottom 0.152: v45.88,4.29 52.07,10.48 v57.15,10.48
PK1_TX  (1 unrouted)
RESET  (via drill 0.33)
  Top 0.152: v23.65,31.27 23.34,31.27 22.54,32.07 SENSORMCU1.29 | v8.57,33.18 7.46,34.29 JP4.1 4.45,34.29 RPUP1.1
  Bottom 0.152: v23.65,31.27 21.75,33.18 v8.57,33.18
RESET1  (via drill 0.33)
  Top 0.152: v37.78,6.99 36.2,6.99 35.88,7.3 35.88,7.78 SERVOMCU.29 | v37.47,5.71 37.47,4.45 37.15,4.13 | JP5.1 43.5,2.54 42.7,1.75 39.53,1.75 37.15,4.13 | 37.15,4.13 RPUP.1
  Bottom 0.152: v37.78,6.99 37.78,5.71 v37.47,5.71
RX_HC  (via drill 0.33)
  Top 0.152: v57.94,13.02 57.94,8.41 55.88,8.41 IC7.24 | v57.31,37.15 58.1,37.94 JP3.1
  Bottom 0.152: v57.94,13.02 57.94,37.15 v57.31,37.15
SCK
  Top 0.152: JP4.2 13.33,34.29 16.19,31.43 16.99,31.43 17.3,31.75 17.62,31.75 SENSORMCU1.17
SCK1  (via drill 0.33)
  Top 0.152: v31.59,11.91 33.18,11.91 SERVOMCU.17 | v40.01,3.17 40.96,3.17 JP5.2
  Bottom 0.152: v31.59,11.91 31.59,3.17 v40.01,3.17
SV1PS
  Top 0.152: 23.5,6.19 24.77,7.46 U1.2 | 23.5,6.19 23.18,5.87 R7.1 | SV1.3 23.65,6.19 23.5,6.19
SV2PS
  Top 0.152: U3.2 6.98,7.62 | 6.98,7.62 6.98,6.67 R15.1 | 6.98,7.62 9.37,7.62 9.53,7.46 9.53,3.81 SV2.3
SV3PS
  Top 0.152: 15.24,6.67 15.24,7.62 17.14,9.53 U5.2 | SV3.3 17.78,3.65 15.24,6.19 15.24,6.67 | 15.24,6.67 R9.1
SV4PS  (via drill 0.33)
  Top 0.152: v28.1,25.88 28.1,24.45 23.97,20.32 22.38,20.32 20.95,21.75 U7.2 20.95,23.65 19.53,25.08 R16.1
  Bottom 0.152: v28.1,25.88 39.37,37.15 SV4.3
SV5PS
  Top 0.152: 14.29,23.5 14.29,20.64 13.02,19.37 U9.2 | 14.29,23.5 14.29,26.67 R11.1 | SV5.3 29.05,41.12 3.65,41.12 3.65,33.5 7.14,30 10.64,30 10.64,23.81 10.95,23.5 14.29,23.5
TARGET_ID
  Top 0.152: U4.2 64.14,26.99 64.29,27.15 64.29,27.78 63.98,28.1 63.34,28.1 63.02,27.78 63.02,24.77 65.88,21.91 75.56,21.91 | 75.56,21.91 75.56,36.2 73.98,37.78 71.75,37.78 71.12,37.15 71.12,36.35 JP6.ID1 | 75.56,21.91 R20.2
TARGET_VBUS/3.2C
  Top 0.152: 67.94,27.62 68.42,28.1 73.98,28.1 75.09,29.21 75.09,34.13 73.02,36.2 JP6.VBUS1 | 67.94,27.62 65.41,25.08 64.77,25.08 U4.6 | 67.94,27.62 67.94,28.42 63.18,28.42 62.71,27.94 62.71,21.59 68.58,21.59 70.17,20 70.17,18.57 71.12,17.62 IC7.96
TX_HC  (via drill 0.33)  (1 unrouted)
  Top 0.152: RPUP2.2 53.98,33.02 53.98,34.61 RPUP3.1 54.13,34.61 v54.13,35.88 | v54.13,37.62 55.56,39.05 JP3.2
  Bottom 0.152: v54.13,37.62 v54.13,35.88
USBD_N  (via drill 0.33)  (1 unrouted)
  Top 0.152: v64.77,26.67 64.77,25.88 U4.1 | v72.39,34.29 72.39,36.2 JP6.D-1
  Bottom 0.152: v72.39,34.29 v64.77,26.67
USBD_P  (via drill 0.33)
  Top 0.152: v63.66,27.46 63.66,25.88 U4.3 | v71.28,35.08 71.75,35.56 JP6.D+1 | v69.85,17.78 69.85,16.83 71.12,16.83 IC7.94
  Bottom 0.152: v71.28,35.08 v63.66,27.46 63.66,23.97 v69.85,17.78
VCC  (via drill 0.33)
  Top 0.152: 60.8,36.51 60.8,36.99 U$1.1 | 60.8,36.51 61.91,35.4 64.45,35.4 R6.2 64.45,35.24 70.64,29.05 70.96,29.05 JP1.VCC | 60.8,36.51 54.77,36.51 | 54.77,36.51 53.34,36.51 50.32,33.5 48.1,33.5 U2.3 | v42.07,6.19 43.5,7.62 JP5.5 54.77,15.08 54.77,36.51 | v32.23,4.45 27.15,9.53 U1.3 26.99,9.68 25.72,10.95 19.53,10.95 19.53,9.68 U5.3 19.37,9.68 14.13,14.92 14.13,16.19 | C9.1 2.54,27.62 | C10.1 4.45,27.62 | 4.45,27.62 5.71,27.62 | 5.71,27.62 6.35,27.62 C3.1 6.35,27.46 7.78,26.04 7.78,22.23 8.09,22.19 | 4.45,27.62 2.54,27.62 | 2.54,27.62 C8.1 | 4.45,27.62 C6.1 | 5.71,27.62 JP4.5 | 8.09,22.19 U9.3 | 8.1,16.19 8.1,22.23 8.09,22.19 | 8.1,16.19 8.1,9.68 U3.3 | 14.13,16.19 14.29,16.35 14.29,17.46 18.57,21.75 U7.3 | 8.1,16.19 14.13,16.19
  Bottom 0.152: v32.23,4.45 35.72,4.45 36.04,4.76 40.64,4.76 v42.07,6.19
